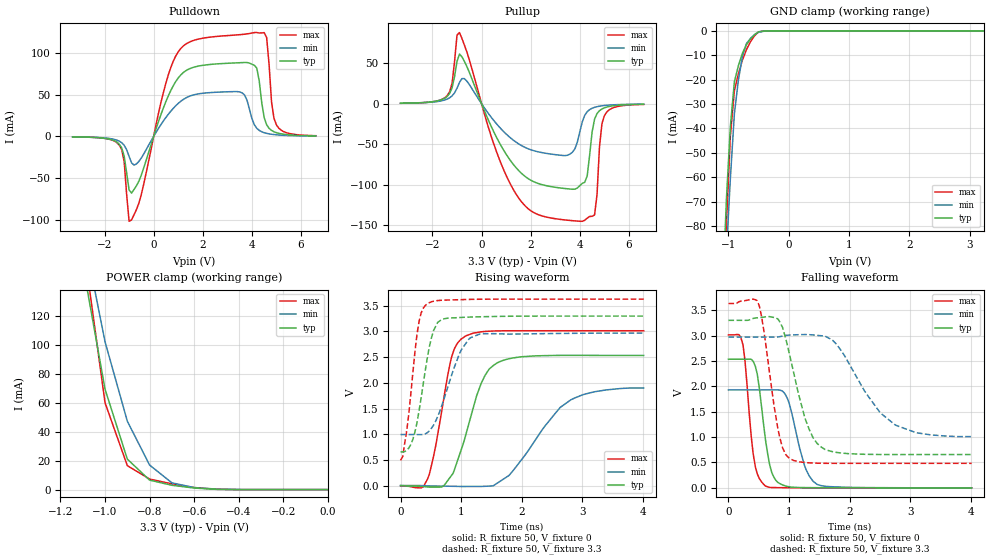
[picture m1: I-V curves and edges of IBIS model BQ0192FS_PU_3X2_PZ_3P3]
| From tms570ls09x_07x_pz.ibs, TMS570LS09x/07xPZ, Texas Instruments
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|IQ0087FS_3X2_3P3; PULLDOWN_OFF
|   Model Cell BQ0192FS_PU_3X2_PZ_3P3
|BQ0192FS_PU_3X2_PZ_3P3
[Model]   BQ0192FS_PU_3X2_PZ_3P3
Model_type   I/O
Polarity   Non-Inverting
Enable   Active-Low
Vinl =  1.25
Vinh =  1.65
Cref =  15.0001pF
Rref =  101.0000M
Vref =  0V
Vmeas =  1.65
C_comp   1.2p   1.2p   1.2p
[Model Spec]
Vinl   1.25   1.12   1.38
Vinh   1.65   1.45   1.75
[Temperature Range]   25   155   -40
[Voltage Range]   3.3   2.97   3.63
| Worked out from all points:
|   slope of the pulldown table from 0 to 0.495 V, typ, clamps not added: 11.9 ohm
|   slope of the pullup table from 0 to 0.495 V, typ, clamps not added: 14.3 ohm
|   GND clamp passes 1 mA (typ) near -0.53 V on its own axis
|   POWER clamp passes 1 mA (typ) near -0.59 V on its own axis
|   rising waveform, R_fixture 50, V_fixture 0: 20-80 % time 399ps typ, 718ps min, 275ps max; typ from 0 V to 2.53 V
|   rising waveform, R_fixture 50, V_fixture 3.3: 20-80 % time 224ps typ, 347ps min, 171ps max; typ from 0.656 V to 3.3 V
|   falling waveform, R_fixture 50, V_fixture 0: 20-80 % time 170ps typ, 243ps min, 138ps max; typ from 2.53 V to 0 V
|   falling waveform, R_fixture 50, V_fixture 3.3: 20-80 % time 342ps typ, 655ps min, 230ps max; typ from 3.3 V to 0.657 V
[POWER_clamp]
|   voltage   I(typ)   I(min)   I(max)
-3.3V     2.375A     2.63A      3.153A
-1.1V     156mA      180.2mA    173.4mA
-1.067V   127.2mA    154.3mA    135.6mA
-1.033V   98.41mA    128.4mA    97.92mA
-1V       69.61mA    102.5mA    60.2mA
-900mV    21.13mA    47.41mA    16.61mA
-800mV    6.576mA    17mA       7.309mA
-700mV    2.999mA    4.688mA    3.99mA
-600mV    1.087mA    1.404mA    1.425mA
-500mV    187uA      358.1uA    203.4uA
0V        311.4pA    5.945nA    272.3pA
[Pulldown]
|   voltage   I(typ)   I(min)   I(max)
-3.3V     -554.3uA   -511.5uA   -526.2uA
-1.4V     -9.291mA   -5.703mA   -10.34mA
-1.2V     -23.68mA   -10.64mA   -30.19mA
-1V       -64.35mA   -24mA      -101.9mA
-600mV    -53.61mA   -29.92mA   -79.98mA
1V        70.16mA    39.6mA     101.5mA
3.5V      88.44mA    53.42mA    122.1mA
4.2V      81.93mA    9.711mA    124.7mA
4.6V      13.96mA    3.646mA    118.8mA
4.8V      7.183mA    2.57mA     41.14mA
5V        4.453mA    1.905mA    13.75mA
6.6V      621.1uA    479.2uA    840.9uA
[Pullup]
|   voltage   I(typ)   I(min)   I(max)
-3.3V     614.6uA    591.9uA    551.1uA
-1.4V     9.028mA    5.738mA    10.01mA
-900mV    61.32mA    26.24mA    87.8mA
1.4V      -78.76mA   -47.33mA   -111.2mA
3.5V      -105mA     -63.56mA   -143.7mA
4.1V      -98.29mA   -22.39mA   -145.1mA
4.3V      -89.13mA   -9.839mA   -141.1mA
4.6V      -19.02mA   -4.469mA   -137.2mA
4.7V      -12.15mA   -3.653mA   -112.5mA
4.8V      -8.616mA   -3.042mA   -53.65mA
5V        -5.089mA   -2.205mA   -14.76mA
6.6V      -663.5uA   -536.5uA   -825.6uA
[GND_clamp]
|   voltage   I(typ)   I(min)   I(max)
-3.3V     -1.947A    -1.623A    -3.254A
-1.1V     -112mA     -127mA     -135.8mA
-1.033V   -69.61mA   -91.63mA   -80.19mA
-966.7mV  -39.23mA   -60.62mA   -43.11mA
-900mV    -20.86mA   -34.02mA   -24.52mA
-833.3mV  -14.26mA   -20.12mA   -17.61mA
-766.7mV  -9.194mA   -10.52mA   -12.01mA
-700mV    -5.668mA   -5.208mA   -7.706mA
-566.7mV  -1.566mA   -1.573mA   -2.055mA
-500mV    -402.3uA   -585.8uA   -459.7uA
-300mV    -821.9nA   -7.17uA    -404.6nA
3.233V    296.5pA    4.008uA    206.9pA
[Ramp]
| variable   typ   min   max
dV/dt_f   1.632013/0.3487527n   1.217272/0.6768432n   1.9423/0.2338758n
dV/dt_r   1.54006/0.4015207n   1.170175/0.7480784n   1.835732/0.2780758n
R_load = 50
[Rising Waveform]
R_fixture = 50
V_fixture = 0
V_fixture_min = 0
V_fixture_max = 0
|   time   V(typ)   V(min)   V(max)
0s        300uV      -880.9nV   -9.822mV
340ps     -15.63mV   -293.8uV   -44.98mV
444ps     -27.35mV   -6.969mV   122.3mV
580ps     -31.8mV    -9.755mV   768.8mV
840ps     194.9mV    -13.95mV   2.49V
1.072ns   966.9mV    -18.2mV    2.91V
1.332ns   1.993V     -17.64mV   2.993V
1.656ns   2.422V     93.12mV    3.013V
2.808ns   2.535V     1.668V     3.014V
4.012ns   2.534V     1.9V       3.014V
[Rising Waveform]
R_fixture = 50
V_fixture = 3.3
V_fixture_min = 2.97
V_fixture_max = 3.63
|   time   V(typ)   V(min)   V(max)
0s        656.3mV    993.4mV    492.9mV
36ps      655.2mV    993.4mV    562.6mV
104ps     687.9mV    993.4mV    1.08V
204ps     901.2mV    993.5mV    2.203V
308ps     1.47V      992.1mV    3.206V
444ps     2.498V     1.03V      3.544V
612ps     3.176V     1.34V      3.602V
972ps     3.272V     2.564V     3.619V
1.152ns   3.281V     2.876V     3.625V
4.012ns   3.3V       2.969V     3.63V
[Falling Waveform]
R_fixture = 50
V_fixture = 0
V_fixture_min = 0
V_fixture_max = 0
|   time   V(typ)   V(min)   V(max)
0s        2.534V     1.93V      3.014V
240ps     2.534V     1.93V      2.817V
408ps     2.494V     1.93V      672.1mV
476ps     2.239V     1.93V      275.2mV
612ps     940.9mV    1.93V      33.73mV
716ps     298mV      1.93V      7.304mV
944ps     36.45mV    1.828V     3.347mV
1.256ns   5.525mV    437.9mV    1.067mV
1.464ns   3.168mV    67.32mV    658.1uV
4.012ns   95.81uV    783uV      -1.864uV
[Falling Waveform]
R_fixture = 50
V_fixture = 3.3
V_fixture_min = 2.97
V_fixture_max = 3.63
|   time   V(typ)   V(min)   V(max)
0s        3.3V       2.97V      3.63V
476ps     3.349V     2.97V      3.686V
580ps     3.363V     2.97V      3.132V
816ps     3.327V     2.972V     1.166V
892ps     3.162V     2.99V      792.6mV
1.024ns   2.543V     3.01V      567.5mV
1.28ns    1.314V     3.021V     497.1mV
1.592ns   757mV      2.989V     483.4mV
2.752ns   655.9mV    1.238V     482.5mV
4.012ns   656.6mV    1.01V      482.2mV
